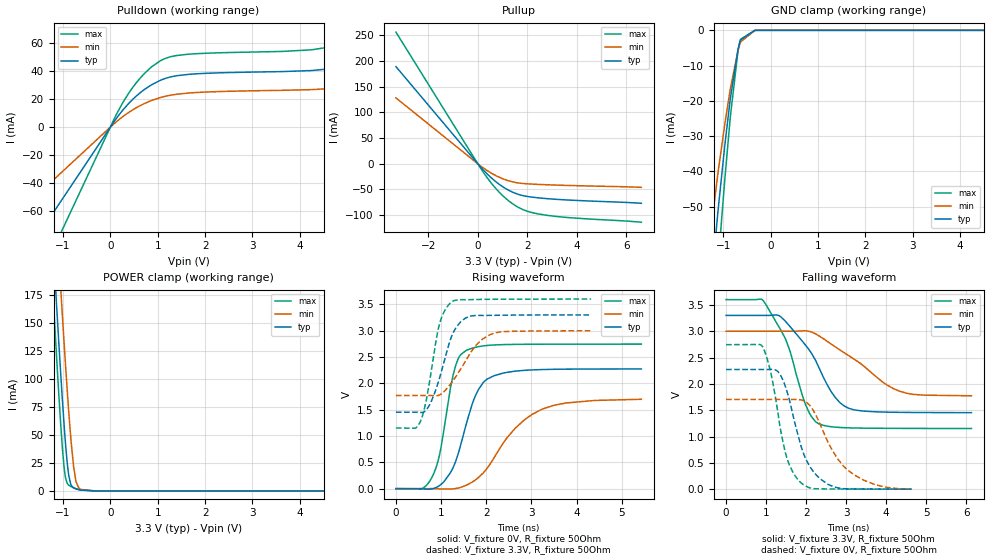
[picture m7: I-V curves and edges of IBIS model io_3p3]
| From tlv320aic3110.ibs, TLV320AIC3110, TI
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|   io_3p3 Model
[Model]   io_3p3
Model_type   I/O
Polarity   Non-Inverting
Enable   Active-High
Vinl = 0.99
Vinh = 2.31
Vmeas = 1.65
Vref = 0
Cref = 10pF
Rref = 50
|   typ   min   max
|   (nom PVT)   (fast PVT)   (slow PVT)
C_comp   1.439e-12   1.410e-12   1.471e-12
| Where nom  PVT is Nominal Process, 3.3V, 27C
|   Fast PVT is Strong Process,  3.6V, -40C
|   Slow PVT is Weak Process,   3V, 125C
[Model spec]
Vinl   0.99   0.90   1.08
Vinh   2.31   2.10   2.52
[Voltage Range]   3.3   3   3.6
|Junction Temperature
[Temperature Range]   27   125   -40
[Pullup Reference]   3.3   3   3.6
[Pulldown Reference]   0   0   0
[Power Clamp Reference]   3.3   3   3.6
[GND Clamp Reference]   0   0   0
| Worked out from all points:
|   slope of the pulldown table from 0 to 0.495 V, typ, clamps not added: 24.1 ohm
|   slope of the pullup table from 0 to 0.495 V, typ, clamps not added: 19.6 ohm
|   POWER clamp passes 1 mA (typ) near -0.65 V on its own axis
|   falling waveform, V_fixture 3.3V, R_fixture 50Ohm: 20-80 % time 881ps typ, 1.31ns min, 670ps max; typ from 3.3 V to 1.45 V
|   rising waveform, V_fixture 0V, R_fixture 50Ohm: 20-80 % time 497ps typ, 951ps min, 339ps max; typ from 0 V to 2.27 V
|   rising waveform, V_fixture 3.3V, R_fixture 50Ohm: 20-80 % time 394ps typ, 572ps min, 299ps max; typ from 1.45 V to 3.3 V
|   falling waveform, V_fixture 0V, R_fixture 50Ohm: 20-80 % time 539ps typ, 806ps min, 416ps max; typ from 2.27 V to 0.002 V
[Pulldown]
|   Voltage   I(typ)   I(min)   I(max)
-3.3V     -167.2mA   -103.4mA   -238.3mA
-142.8mV  -7.234mA   -4.473mA   -10.31mA
153mV     7.459mA    4.581mA    10.75mA
462mV     19.5mA     12.14mA    27.88mA
855mV     29.92mA    18.83mA    42.57mA
1.164V    34.82mA    22.06mA    49.12mA
1.827V    38.11mA    24.74mA    52.46mA
4.713V    41.95mA    27.72mA    57.69mA
5.409V    48.17mA    31.48mA    67.49mA
5.732V    53.67mA    34.85mA    76.03mA
6.33V     70.26mA    45.18mA    101.4mA
6.6V      81.12mA    52.02mA    117.9mA
[GND Clamp]
|   Voltage   I(typ)   I(min)   I(max)
-3.3V     -1.774A    -1.53A     -1.959A
-1.482V   -105.7mA   -80.68mA   -134.7mA
-1.116V   -51.96mA   -40.93mA   -67.47mA
-1.104V   -50.33mA   -39.72mA   -65.37mA
-966.9mV  -32.6mA    -26.57mA   -42.24mA
-851.4mV  -19.43mA   -16.67mA   -24.65mA
-690mV    -5.546mA   -5.78mA    -6.021mA
-660mV    -3.846mA   -4.324mA   -3.871mA
-636mV    -2.74mA    -3.325mA   -2.546mA
-330mV    -1.064uA   -10.19uA   -112.4nA
6.6V      0A         0A         0A
[Pullup]
|   Voltage   I(typ)   I(min)   I(max)
-3.3V     189.2mA    128.2mA    256.5mA
181.2mV   -9.972mA   -6.723mA   -13.56mA
492mV     -25.14mA   -16.79mA   -34.41mA
786mV     -37.23mA   -24.59mA   -51.33mA
1.275V    -52.45mA   -33.81mA   -73.46mA
1.566V    -58.58mA   -37.05mA   -83.09mA
1.881V    -62.82mA   -38.83mA   -90.58mA
2.201V    -65.24mA   -39.78mA   -95.4mA
2.798V    -68.14mA   -41.09mA   -100.7mA
3.633V    -70.8mA    -42.41mA   -105mA
6.6V      -77.12mA   -46.09mA   -114mA
[POWER Clamp]
|   Voltage   I(typ)   I(min)   I(max)
-3.3V     1.91A      1.953A     1.91A
-1.264V   261.7mA    338.2mA    217.1mA
-1.151V   177.4mA    254.6mA    131.1mA
-1.05V    106mA      182.5mA    60.61mA
-1.013V   81.58mA    156.9mA    38.48mA
-960mV    49.38mA    121.3mA    15.21mA
-877.8mV  13.67mA    70.33mA    5.079mA
-777mV    2.69mA     22.17mA    2.882mA
-732mV    1.852mA    9.951mA    2.151mA
-633mV    810.6uA    1.359mA    886.9uA
-330mV    1.425uA    4.902uA    317.2nA
6.6V      0A         0A         0A
[Ramp]
R_load = 50
|   typ   min   max
dV/dt_r   1.36423/4.95871e-10   1.02263/9.5737e-10   1.64702/3.37236e-10
dV/dt_f   1.10913/8.80496e-10   0.73866/1.31738e-09   1.46873/6.69949e-10
[Falling Waveform]
V_fixture = 3.3V
V_fixture_min = 3V
V_fixture_max = 3.6V
R_fixture = 50Ohm
|   Time   V(typ)   V(min)   V(max)
0s        3.3V       3V         3.6V
939ps     3.3V       3V         3.572V
1.363ns   3.277V     3V         3.028V
1.569ns   3.115V     3V         2.685V
1.984ns   2.738V     3.007V     1.614V
2.311ns   2.327V     2.917V     1.244V
2.732ns   1.74V      2.702V     1.179V
3.066ns   1.536V     2.536V     1.165V
4.337ns   1.46V      1.861V     1.155V
6.134ns   1.453V     1.774V     1.153V
[Rising Waveform]
V_fixture = 0V
V_fixture_min = 0V
V_fixture_max = 0V
R_fixture = 50Ohm
|   Time   V(typ)   V(min)   V(max)
0s        1.257nV    20.5nV     828.8pV
789ps     -5.997mV   600.2uV    201.2mV
967ps     60.03mV    -4.8mV     649.2mV
1.32ns    511.9mV    2.443mV    2.331V
1.556ns   1.224V     63.81mV    2.625V
1.83ns    1.885V     213.8mV    2.697V
2.176ns   2.144V     592.8mV    2.728V
2.64ns    2.231V     1.147V     2.739V
3.238ns   2.261V     1.51V      2.742V
5.432ns   2.273V     1.697V     2.745V
[Rising Waveform]
V_fixture = 3.3V
V_fixture_min = 3V
V_fixture_max = 3.6V
R_fixture = 50Ohm
|   Time   V(typ)   V(min)   V(max)
0s        1.451V     1.769V     1.152V
422ps     1.452V     1.769V     1.147V
537ps     1.447V     1.769V     1.265V
733ps     1.573V     1.769V     1.972V
968ps     2.11V      1.78V      3.137V
1.265ns   2.955V     2.052V     3.562V
1.541ns   3.24V      2.423V     3.587V
1.808ns   3.29V      2.755V     3.592V
2.172ns   3.291V     2.954V     3.596V
4.32ns    3.299V     2.998V     3.6V
[Falling Waveform]
V_fixture = 0V
V_fixture_min = 0V
V_fixture_max = 0V
R_fixture = 50Ohm
|   Time   V(typ)   V(min)   V(max)
0s        2.274V     1.705V     2.745V
918ps     2.274V     1.705V     2.701V
1.128ns   2.274V     1.705V     2.179V
1.381ns   2.138V     1.704V     1.055V
1.585ns   1.689V     1.705V     457.6mV
1.882ns   795.6mV    1.695V     116mV
2.356ns   195mV      1.223V     6.543mV
3.012ns   7.451mV    383.1mV    2.598mV
3.73ns    2.928mV    86mV       1.508mV
4.634ns   1.589mV    3.69mV     761.8uV
